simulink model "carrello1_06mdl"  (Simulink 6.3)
settings: Solver=ode45  SolverMode=SingleTasking  StartTime=0.0  StopTime=10.0  RelTol=1e-6  AbsTol=1e-7
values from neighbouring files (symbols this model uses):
  A_dis = 1*10*cm    (= 0.1)    [carrello_06.m]
  b1 = 2*1500*N/(m/sec)    (= 3000)    [carrello_06.m]
  b2 = 2*1500*N/(m/sec)    (= 3000)    [carrello_06.m]
  F = 0    [carrello_06.m]
  Freq_dis = 1*5*rad/sec    (= 5)    [carrello_06.m]
  K = 0.8*1800*N/cm    (= 144000)    [carrello_06.m]
  Kp = 2*1800*N/cm    (= 360000)    [carrello_06.m]
  Ma = 3850*Kg    (= 3850)    [carrello_06.m]
  Mag = Ma*g    (= 37768.5)    [carrello_06.m]
  mr = 2*134*Kg+524*Kg    (= 792)    [carrello_06.m]
  mrg = mr*g    (= 7769.52)    [carrello_06.m]
  X_12_0 = -Mag/K    (= -0.26228125)    [carrello_06.m]
  X_20_0 = -(Mag+mrg)/Kp    (= -0.1264945)    [carrello_06.m]
libraries: simulink x5

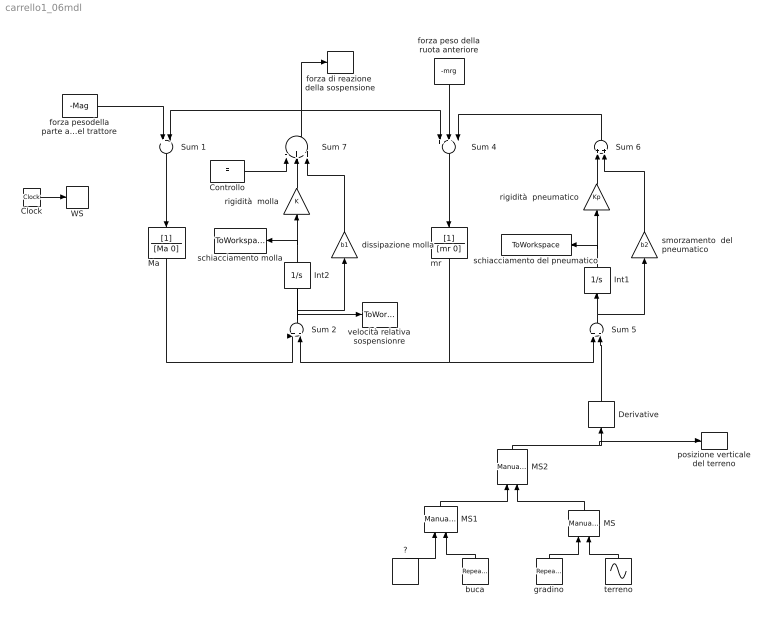
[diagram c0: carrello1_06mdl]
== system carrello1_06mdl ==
  "?" : DiscretePulseGenerator  Orientation=up  PulseType=Time based  Amplitude=0  Period=1  PulseWidth=50
  Clock : Clock
  Controllo : Constant  Value=F
  Derivative : Derivative  Orientation=up
  Int1 : Integrator  Orientation=up  InitialCondition=X_20_0
  Int2 : Integrator  Orientation=up  InitialCondition=X_12_0
  MS : simulink/Signal Routing/Manual Switch  Orientation=up  sw=1  action=0
  MS1 : simulink/Signal Routing/Manual Switch  Orientation=up  sw=1  action=0
  MS2 : simulink/Signal Routing/Manual Switch  Orientation=up  sw=0  action=0
  Ma : TransferFcn  Orientation=down  Denominator=[Ma 0]
  Sum 1 : Sum  Orientation=down  Inputs=+-
  Sum 2 : Sum  Orientation=up  Inputs=+-
  Sum 4 : Sum  Orientation=down  Inputs=++-
  Sum 5 : Sum  Orientation=up  Inputs=+-
  Sum 6 : Sum  Orientation=up
  Sum 7 : Sum  Orientation=up  Inputs=-++
  WS : ToWorkspace  VariableName=t  SampleTime=-1  SaveFormat=Array
  buca : simulink/Sources/Repeating Sequence  Orientation=up  rep_seq_t=[0 1 1.01 3 3.01 10]  rep_seq_y=[0 0 -0.1 -0.1 0 0]
  dissipazione molla : Gain  Orientation=up  Gain=b1
  forza di reazione  della sospensione : ToWorkspace  VariableName=R  SampleTime=-1  SaveFormat=Array
  forza peso della ruota anteriore : Constant  Orientation=down  Value=-mrg
  forza pesodella parte anteriore del trattore : Constant  Value=-Mag
  gradino : simulink/Sources/Repeating Sequence  Orientation=up  rep_seq_t=[0 1 1.01 3 3.01 10]  rep_seq_y=[0 0 0.1 0.1 0 0]
  mr : TransferFcn  Orientation=down  Denominator=[mr 0]
  posizione verticale del terreno : ToWorkspace  VariableName=Xs  SampleTime=-1  SaveFormat=Array
  rigidità  molla : Gain  Orientation=up  Gain=K
  rigidità  pneumatico : Gain  Orientation=up  Gain=Kp
  schiacciamento del pneumatico : ToWorkspace  VariableName=X_20  SampleTime=-1  SaveFormat=Array
  schiacciamento molla : ToWorkspace  VariableName=X_12  SampleTime=-1  SaveFormat=Array
  smorzamento  del pneumatico : Gain  Orientation=up  Gain=b2
  terreno : Sin  Orientation=up  Amplitude=A_dis  Frequency=Freq_dis  SampleTime=0
  velocità relativa sospensionre : ToWorkspace  VariableName=vel_rel  SampleTime=-1  SaveFormat=Array
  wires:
  forza pesodella parte anteriore del trattore/1 -> Sum 1/1
  Sum 1/1 -> Ma/1
  forza peso della ruota anteriore/1 -> Sum 4/2
  Sum 4/1 -> mr/1
  mr/1 -> Sum 5/1, Sum 2/2
  Int1/1 -> rigidità  pneumatico/1, schiacciamento del pneumatico/1
  Sum 5/1 -> Int1/1, smorzamento  del pneumatico/1
  rigidità  pneumatico/1 -> Sum 6/1
  smorzamento  del pneumatico/1 -> Sum 6/2
  Clock/1 -> WS/1
  Sum 7/1 -> Sum 1/2, forza di reazione  della sospensione/1, Sum 4/1
  Sum 6/1 -> Sum 4/3
  Sum 2/1 -> velocità relativa sospensionre/1, Int2/1, dissipazione molla/1
  Int2/1 -> rigidità  molla/1, schiacciamento molla/1
  terreno/1 -> MS/2
  gradino/1 -> MS/1
  MS1/1 -> MS2/1
  MS/1 -> MS2/2
  "?"/1 -> MS1/1
  buca/1 -> MS1/2
  MS2/1 -> posizione verticale del terreno/1, Derivative/1
  dissipazione molla/1 -> Sum 7/3
  rigidità  molla/1 -> Sum 7/2
  Controllo/1 -> Sum 7/1
  Derivative/1 -> Sum 5/2
  Ma/1 -> Sum 2/1
